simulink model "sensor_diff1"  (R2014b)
settings: Solver=ode45  StartTime=0.0  StopTime=10.0  RelTol=1e-3
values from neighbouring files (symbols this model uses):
  b = fliplr(a)    [lattice_11.m]    (also in sensor_diff_1.m = firpm(N,[0,0.5]*2, [0, pi], 'differentiator'); sgolay_1.m = sgolay(k,f))
  delay = N*Ts/2    (= 0.0165)    [sensor_diff_1.m]
  fs = 1000    [abtast_fir_1.m]    (also in abtast_fir_2.m; abtast_fir_3.m; abtast_fir_4.m; hilbert_filter_1.m)
  fsig = 100    [sensor_diff_1.m]    (also in abtast_rate_1.m; ad_test_12.m = ',num2str(fsig),'; ad_test_2.m = ',num2str(fsig),'; ad_test_3.m = ',num2str(fsig),')
  Ts = 1/fs    (= 0.001)    [abtast_fir_1.m]    (also in abtast_fir_2.m; abtast_fir_3.m; abtast_fir_4.m; hilbert_filter_1.m)
libraries: dsparch4 x1

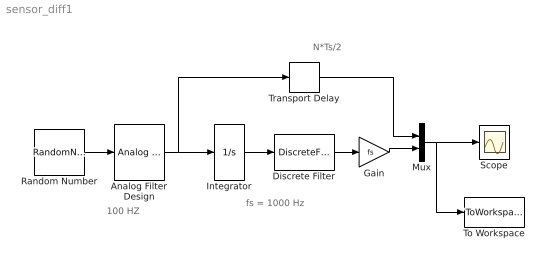
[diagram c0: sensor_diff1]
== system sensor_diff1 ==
  note: N*Ts/2
  note: fs = 1000 Hz
  note: 100 HZ
  Analog Filter Design : dsparch4/Analog Filter Design  method=Butterworth  filttype=Lowpass  N=8  Wlo=2*pi*fsig  Whi=80  Rp=2  Rs=40
  Discrete Filter : DiscreteFilter  Numerator=b  Denominator=1  SampleTime=Ts
  Gain : Gain  Gain=fs
  Integrator : Integrator
  Mux : Mux  Inputs=2
  Random Number : RandomNumber  SampleTime=1e-4
  Scope : Scope
  To Workspace : ToWorkspace  VariableName=y  SaveFormat=Timeseries  SampleTime=-1
  Transport Delay : TransportDelay  DelayTime=delay
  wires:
  Random Number/1 -> Analog Filter Design/1
  Discrete Filter/1 -> Gain/1
  Integrator/1 -> Discrete Filter/1
  Analog Filter Design/1 -> Transport Delay/1, Integrator/1
  Gain/1 -> Mux/2
  Mux/1 -> To Workspace/1, Scope/1
  Transport Delay/1 -> Mux/1
